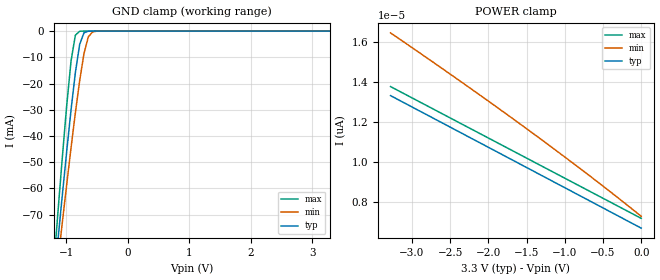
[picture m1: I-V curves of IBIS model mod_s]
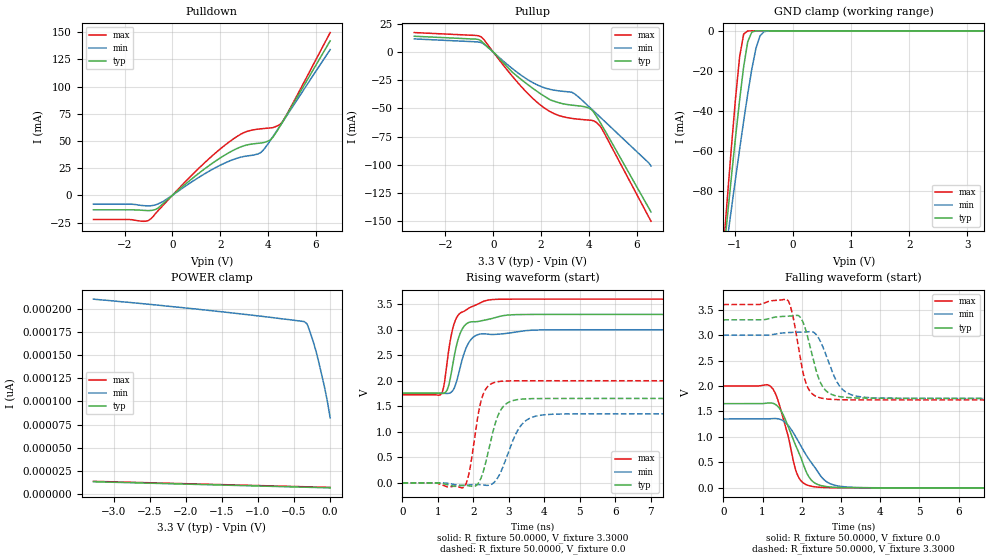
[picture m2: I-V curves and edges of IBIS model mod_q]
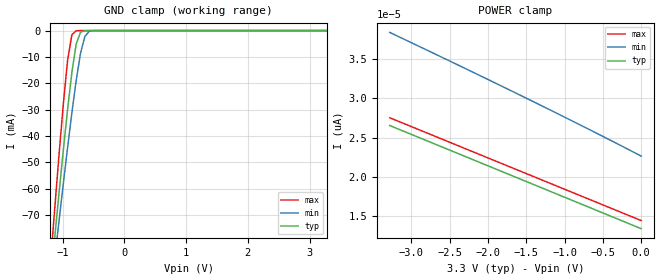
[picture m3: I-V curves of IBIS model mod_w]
| IBIS (I/O, Buffer, Information, Specification) Model, officially
| electronic behavioral standard for Buffer structures of digital pins.
[IBIS ver]  4.0
[File name] m95m02ef_3v3_dfn8.ibs
[File Rev]  1.0
[Date]   21 Jan 2026
[Source]   CAD & Design Services (Catania) - STMicroelectronics
[Notes]
   (Note1)  This IBIS model includes DFN8 Package parasitic data
   (Note2)  This IBIS model considers: VCC=3.30(TYP), 3.00(MIN), 3.60(MAX)
   (Note3)  This IBIS model has some Notes about the non-monotonicity
   of the I-V curves, but they are not indicative of problems
   inside the model;
[Disclaimer]
   Customers are solely responsible for all aspects of their
   own product designs or applications using this IBIS Model.
   STMicroelectronics assumes no liability for Custmer Designs
   and applications associated to this IBIS Model.
   In the use of this IBIS Model Customer shall not modify,
   disassemble, alter this Model in whole or in part.
   If Customers do not accept these terms, the IBIS Model
   may not be used. For any problems or modifications please
   contact STMicroelectronics (www.st.com).
[Copyright] (c) 2026 STMicroelectronics
|   Component M95M02EF
[Component] M95M02EF
[Manufacturer] STMicroelectronics
[Package]
| variable   typ   min   max
R_pkg   0.0   0.0   0.0
L_pkg   0.0H   0.0H   0.0H
C_pkg   0.0F   0.0F   0.0F
[Pin]  signal_name   model_name   R_pin   L_pin   C_pin
1   SN   mod_s   0.0   0.0   0.0
2   Q   mod_q   0.0   0.0   0.0
3   WN   mod_w   0.0   0.0   0.0
4   GND   GND   0.0   0.0   0.0
5   D   mod_d   0.0   0.0   0.0
6   C   mod_c   0.0   0.0   0.0
7   H   mod_h   0.0   0.0   0.0
8   VCC   POWER   0.0   0.0   0.0
[Package Model]  182694_DFN8   | also called 182694_MLP_2x3
[Define Package Model]  182694_DFN8
[Manufacturer]  STMicroelectronics
[OEM]  STMicroelectronics
[Description]  8 pin MLP 2x3
[Number Of Pins]  8
[Pin Numbers]
|Pin Num   Terminal Name
1   | net1
2   | net2
3   | net3
4   | net4_GND
5   | net5
6   | net6
7   | net7
8   | net8_VDD
[Model Data]
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[End Model Data]
[End Package Model]
| Models and submodels in the file (6): mod_s (Input), mod_q (I/O), mod_w (Input), mod_d (Input), mod_c (Input), mod_h (Input)
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|   Model mod_s
[Model]   mod_s
Model_type Input
Vinl   =   0.990V
Vinh   =   2.310V
C_comp   3.207pF   2.950pF   3.586pF
[Temperature Range]  25.0000   85.0000   -40.0000
[Voltage Range]   3.3000V   3.0000V   3.6000V
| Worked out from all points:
|   GND clamp passes 1 mA (typ) near -0.72 V on its own axis
[GND_clamp]
|Voltage   I(typ)   I(min)   I(max)
-3.3V     -639.2mA   -563.1mA   -760.8mA
-1.2V     -96.21mA   -101.8mA   -89.25mA
-1.13V    -79.02mA   -87.14mA   -68.17mA
-1.06V    -62.12mA   -72.63mA   -47.66mA
-990mV    -45.69mA   -58.38mA   -28.24mA
-920mV    -30.02mA   -44.49mA   -11.36mA
-850mV    -15.84mA   -31.19mA   -1.554mA
-780mV    -5.062mA   -18.9mA    -59.9uA
-710mV    -636.4uA   -8.601mA   -1.855uA
-640mV    -45.53uA   -2.227mA   -57.01nA
-570mV    -3.005uA   -303.9uA   -1.764nA
3.28V     6.672pA    17.15pA    6.56pA
[POWER_clamp]
|Voltage   I(typ)   I(min)   I(max)
-3.28V    13.31pA    16.43pA    13.76pA
-2.28V    11.3pA     13.79pA    11.76pA
-1.44V    9.611pA    11.5pA     10.08pA
-640mV    8.001pA    9.217pA    8.48pA
0V        6.712pA    7.302pA    7.2pA
|   Model mod_q
[Model]   mod_q
Model_type I/O
Polarity   Non-Inverting
Enable   Active-Low
Vinl   =   0.990V
Vinh   =   1.450V
Vmeas  =   1.650V
Cref   =   30pF
C_comp   3.856pF   3.517pF   4.038pF
[Temperature Range]  25.0000   85.0000   -40.0000
[Voltage Range]   3.3000V   3.0000V   3.6000V
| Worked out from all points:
|   slope of the pulldown table from 0 to 0.495 V, typ, clamps not added: 52.8 ohm
|   slope of the pullup table from 0 to 0.495 V, typ, clamps not added: 44.4 ohm
|   GND clamp passes 1 mA (typ) near -0.72 V on its own axis
|   rising waveform, R_fixture 50.0000, V_fixture 3.3000: 20-80 % time 314ps typ, 340ps min, 305ps max; typ from 1.76 V to 3.3 V
|   rising waveform, R_fixture 50.0000, V_fixture 0.0: 20-80 % time 374ps typ, 490ps min, 281ps max; typ from 0 V to 1.65 V
|   falling waveform, R_fixture 50.0000, V_fixture 0.0: 20-80 % time 513ps typ, 661ps min, 385ps max; typ from 1.65 V to 0 V
|   falling waveform, R_fixture 50.0000, V_fixture 3.3000: 20-80 % time 335ps typ, 413ps min, 276ps max; typ from 3.3 V to 1.76 V
[Pulldown]
|Voltage   I(typ)   I(min)   I(max)
-3.3V     -13.24mA   -8.114mA   -22.15mA
-1.7V     -13.27mA   -8.123mA   -22.33mA
-1V       -13.97mA   -9.639mA   -23.14mA
-600mV    -11.76mA   -7.819mA   -14.18mA
900mV     16.7mA     13.64mA    20.44mA
2.1V      35.73mA    28.74mA    44.38mA
3V        45.61mA    35.77mA    57.72mA
3.7V      48.11mA    39.39mA    61.15mA
4.1V      50.97mA    50.53mA    61.95mA
4.4V      59.9mA     60.35mA    63.97mA
4.6V      67.1mA     67.02mA    67.59mA
6.6V      142mA      133.9mA    149.6mA
[Pullup]
|Voltage   I(typ)   I(min)   I(max)
-3.3V     13.98mA    11.62mA    17.25mA
-800mV    11.56mA    9.122mA    14.78mA
-500mV    9.702mA    8.372mA    13.36mA
1V        -21.45mA   -18mA      -26.51mA
2V        -37.34mA   -30.63mA   -47.47mA
2.6V      -44.05mA   -34.05mA   -55.19mA
3.3V      -47.23mA   -35.85mA   -58.95mA
3.8V      -48.45mA   -44.36mA   -60.08mA
4.1V      -50.97mA   -50.32mA   -60.58mA
4.3V      -56.47mA   -54.32mA   -62.25mA
4.5V      -63.47mA   -58.32mA   -66.55mA
6.6V      -142mA     -101.1mA   -150.2mA
[GND_clamp]
|Voltage   I(typ)   I(min)   I(max)
-3.3V     -758.5mA   -596.9mA   -944.4mA
-1.2V     -113.1mA   -119mA     -109.3mA
-1.13V    -92.65mA   -103.7mA   -83.15mA
-1.06V    -72.59mA   -88.63mA   -57.71mA
-920mV    -34.54mA   -59.15mA   -13.02mA
-850mV    -17.85mA   -44.98mA   -1.616mA
-780mV    -5.439mA   -31.48mA   -60.01uA
-710mV    -645.3uA   -19.12mA   -1.855uA
-640mV    -45.58uA   -8.894mA   -57.01nA
-570mV    -3.005uA   -2.55mA    -1.764nA
-500mV    -197.3nA   -431.8uA   -57.18pA
3.28V     6.672pA    285.1pA    6.56pA
[POWER_clamp]
|Voltage   I(typ)   I(min)   I(max)
-3.28V    13.31pA    210.2pA    13.76pA
-1.84V    10.42pA    199.4pA    10.88pA
-360mV    7.438pA    186pA      7.92pA
-320mV    7.357pA    183.5pA    7.84pA
-280mV    7.277pA    175.1pA    7.76pA
-240mV    7.196pA    165.7pA    7.68pA
-200mV    7.115pA    155.3pA    7.6pA
-160mV    7.035pA    142.9pA    7.52pA
-80mV     6.874pA    116pA      7.36pA
-40mV     6.793pA    100.6pA    7.28pA
0V        6.712pA    82.2pA     7.2pA
[Ramp]
| variable   typ   min   max
dV/dt_r   0.9923/0.4293n   0.8116/0.5411n   1.2002/0.3437n
dV/dt_f   0.9242/0.3840n   0.7466/0.4456n   1.1240/0.3268n
R_load = 50.0000
[Rising Waveform]
R_fixture= 50.0000
V_fixture= 3.3000
V_fixture_min= 3.0000
V_fixture_max= 3.6000
|time   V(typ)   V(min)   V(max)
0s        1.759V     1.756V     1.727V
1.09ns    1.754V     1.756V     1.739V
1.17ns    1.758V     1.754V     1.911V
1.29ns    1.878V     1.753V     2.53V
1.39ns    2.206V     1.786V     2.943V
1.51ns    2.653V     1.952V     3.216V
1.67ns    2.995V     2.382V     3.343V
1.87ns    3.143V     2.748V     3.423V
2.33ns    3.19V      2.919V     3.568V
10ns      3.3V       3V         3.6V
[Rising Waveform]
R_fixture= 50.0000
V_fixture= 0.0
V_fixture_min= 0.0
V_fixture_max= 0.0
|time   V(typ)   V(min)   V(max)
0s        4.159nV    176.8nV    3.059nV
1.74ns    -46.84mV   -52.62mV   -78.72mV
1.89ns    -58.21mV   -40.28mV   235.5mV
2.23ns    122.7mV    -38.19mV   1.643V
2.39ns    525.1mV    -48.77mV   1.878V
2.61ns    1.155V     27.96mV    1.971V
2.85ns    1.503V     343.6mV    1.994V
3.27ns    1.634V     1.054V     2V
3.75ns    1.652V     1.306V     2.001V
10ns      1.654V     1.353V     2.001V
[Falling Waveform]
R_fixture= 50.0000
V_fixture= 0.0
V_fixture_min= 0.0
V_fixture_max= 0.0
|time   V(typ)   V(min)   V(max)
0s        1.654V     1.353V     2.001V
1.23ns    1.667V     1.36V      1.975V
1.35ns    1.627V     1.361V     1.812V
1.49ns    1.491V     1.332V     1.468V
1.87ns    787mV      971.7mV    293.1mV
2.01ns    526.4mV    778.6mV    114.6mV
2.21ns    184.6mV    532.4mV    37.57mV
2.61ns    27.03mV    133.4mV    5.716mV
3.09ns    4.3mV      21.03mV    685.1uV
10ns      36.57nV    231.2nV    -16.71nV
[Falling Waveform]
R_fixture= 50.0000
V_fixture= 3.3000
V_fixture_min= 3.0000
V_fixture_max= 3.6000
|time   V(typ)   V(min)   V(max)
0s        3.3V       3V         3.6V
1.62ns    3.37V      3.049V     3.702V
1.76ns    3.378V     3.053V     3.424V
1.94ns    3.369V     3.057V     2.645V
2.1ns     3.104V     3.063V     2.072V
2.32ns    2.436V     3.046V     1.816V
2.48ns    2.062V     2.87V      1.766V
2.94ns    1.795V     2.027V     1.732V
3.4ns     1.766V     1.801V     1.728V
10ns      1.759V     1.756V     1.727V
|   Model mod_w
[Model]   mod_w
Model_type Input
Vinl   =   0.990V
Vinh   =   2.310V
C_comp   3.207pF   2.950pF   3.586pF
[Temperature Range]  25.0000   85.0000   -40.0000
[Voltage Range]   3.3000V   3.0000V   3.6000V
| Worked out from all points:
|   GND clamp passes 1 mA (typ) near -0.72 V on its own axis
[GND_clamp]
|Voltage   I(typ)   I(min)   I(max)
-3.3V     -639.2mA   -563.1mA   -760.8mA
-1.2V     -96.21mA   -101.8mA   -89.26mA
-1.13V    -79.02mA   -87.14mA   -68.17mA
-1.06V    -62.12mA   -72.63mA   -47.66mA
-990mV    -45.69mA   -58.38mA   -28.24mA
-920mV    -30.02mA   -44.49mA   -11.36mA
-850mV    -15.84mA   -31.19mA   -1.56mA
-780mV    -5.066mA   -18.9mA    -62.28uA
-710mV    -639.4uA   -8.604mA   -2.115uA
-640mV    -46.36uA   -2.229mA   -66.31nA
-570mV    -3.089uA   -305.3uA   -2.053nA
3.28V     13.28pA    24.04pA    13.12pA
[POWER_clamp]
|Voltage   I(typ)   I(min)   I(max)
-3.28V    26.53pA    38.41pA    27.52pA
-1.44V    19.15pA    29.74pA    20.16pA
-680mV    16.1pA     26.03pA    17.12pA
0V        13.37pA    22.63pA    14.4pA
